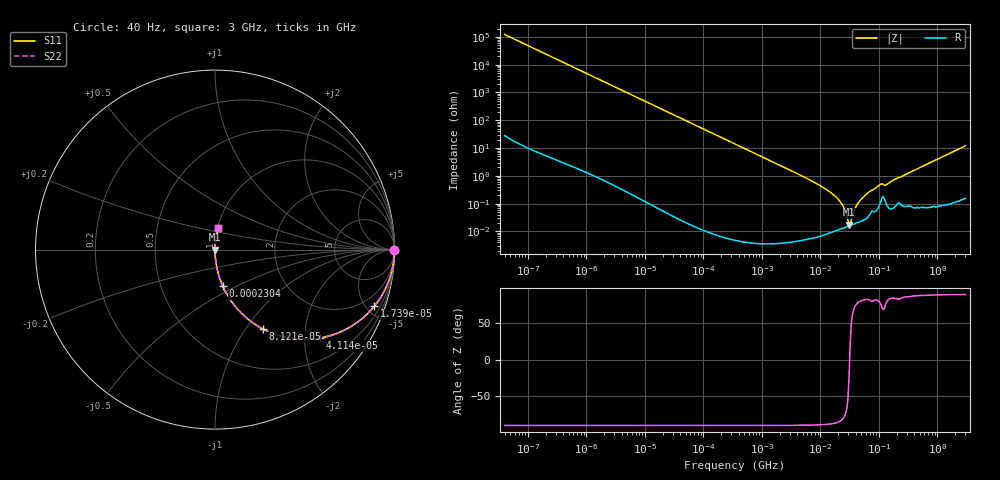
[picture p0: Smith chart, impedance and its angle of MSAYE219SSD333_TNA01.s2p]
! MSAYE219SSD333_TNA01  S-PARAMETER MODEL  ( General Type )
! Model Generated by TAIYO YUDEN Corporation (http://www.ty-top.com)
! Version 2.0
! TAIYO YUDEN Control No. 031016
! Copyright(c) 2003 TAIYO YUDEN CO.,LTD. All Rights Reserved.
! Product Description (link to TY-COMPAS)
! https://ds.yuden.co.jp/TYCOMPAS/or/detail?pn=MSAYE219SSD333KTNA01&u=M
! Products Name : Multilayer Ceramic Capacitors
! Characteristics :
!  Capacitance : 0.033 uF , Rated Voltage : 16V
!  Case Size : 2.0 x 1.25 / 0.079 x 0.049 [mm/inch] , Thickness : 0.85 / 0.033 [mm/inch]
!  (Conditions: Temperature = 25 degC , DC Bias Current/Voltage = 0A / 0V)
! External Node Assignments :
!  1  o---| |---o  2
! GND o---------o GND
! Frequency Range : 40Hz  -  3GHz  [ 401 STEP ]
# MHz S RI R 50
! Freq[MHz].  S11 Real  S11 Imag  S21 Real  S21 Imag  S12 Real  S12 Imag  S22 Real  S22 Imag
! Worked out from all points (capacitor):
!   401 points, 40 Hz to 3 GHz, reference 50 ohm
!   read as one part in series: C = 32.5 nF near 44 Hz
!   lowest |Z| = 17.3 mohm at 30.81 MHz (marker M1)
!   series resonance near 31.54 MHz, so ESL is about 780 pH
!   S11 on the Smith chart (normalised r, x): 40 Hz: open; 17.39 kHz: 1.00, -5.63; 41.14 kHz: 1.00, -2.38; 81.21 kHz: 1.00, -1.21; 230.4 kHz: 1.00, -0.43; 3 GHz: 1.00, +0.24
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4e-05  1 -0.000817  8.54e-07 0.000817  8.54e-07 0.000817  1 -0.000817
0.000834  0.9997 -0.017  0.000295 0.017  0.000295 0.017  0.9997 -0.017
0.004886  0.9901 -0.0988  0.00988 0.0988  0.00988 0.0988  0.9901 -0.0988
0.017386  0.888 -0.3153  0.112 0.3153  0.112 0.3153  0.888 -0.3153
0.041141  0.5862 -0.4924  0.4138 0.4924  0.4138 0.4924  0.5862 -0.4924
0.081206  0.2667 -0.4421  0.7333 0.4421  0.7333 0.4421  0.2667 -0.4421
0.133706  0.1183 -0.3229  0.8817 0.3229  0.8817 0.3229  0.1183 -0.3229
0.230357  0.0433 -0.2034  0.9567 0.2034  0.9567 0.2034  0.0433 -0.2034
0.362475  0.018 -0.1326  0.982 0.1326  0.982 0.1326  0.018 -0.1326
1.178032  0.00176 -0.0414  0.9982 0.0414  0.9982 0.0414  0.00176 -0.0414
7.222098  9.77e-05 -0.00641  0.9999 0.00641  0.9999 0.00641  9.77e-05 -0.00641
13.01976  9.09e-05 -0.0031  0.9999 0.0031  0.9999 0.0031  9.09e-05 -0.0031
19.57906  0.000113 -0.00153  0.9999 0.00153  0.9999 0.00153  0.000113 -0.00153
24.56009  0.000133 -0.000772  0.9999 0.000772  0.9999 0.000772  0.000133 -0.000772
29.4429  0.000153 -0.000213  0.9998 0.000213  0.9998 0.000213  0.000153 -0.000213
30.80834  0.000158 -7.05e-05  0.9998 7.05e-05  0.9998 7.05e-05  0.000158 -7.05e-05
33.73212  0.000167 0.000203  0.9998 -0.000203  0.9998 -0.000203  0.000167 0.000203
42.31378  0.00021 0.000905  0.9998 -0.000905  0.9998 -0.000905  0.00021 0.000905
55.54024  0.000265 0.00181  0.9997 -0.00181  0.9997 -0.00181  0.000265 0.00181
104.7695  0.00106 0.00474  0.9989 -0.00474  0.9989 -0.00474  0.00106 0.00474
150.5692  0.000701 0.00563  0.9993 -0.00563  0.9993 -0.00563  0.000701 0.00563
3000  0.0158 0.1183  0.9842 -0.1183  0.9842 -0.1183  0.0158 0.1183
